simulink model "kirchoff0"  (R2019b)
settings: Solver=ode23s  StartTime=0.0  StopTime=0.01  RelTol=1e-3  EnableMultiTasking=on
libraries: fl_lib x9, nesl_utility x5, powerlib x1

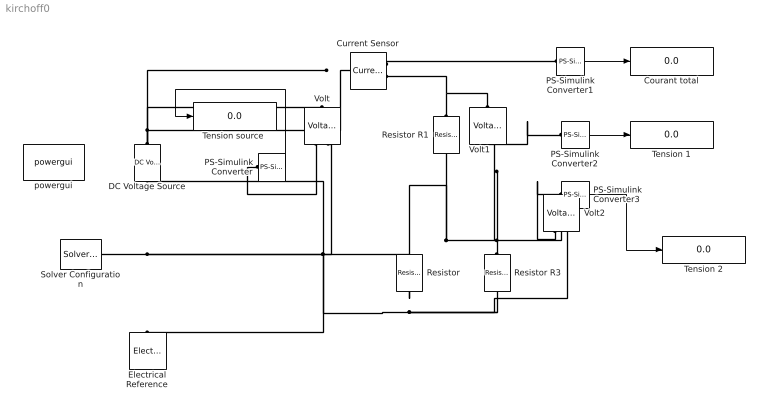
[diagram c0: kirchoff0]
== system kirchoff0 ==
  Courant total : Display
  Current Sensor : fl_lib/Electrical/Electrical Sensors/Current Sensor
  DC Voltage Source : fl_lib/Electrical/Electrical Sources/DC Voltage Source  v0=10 V
  Electrical Reference : fl_lib/Electrical/Electrical Elements/Electrical Reference
  PS-Simulink Converter : nesl_utility/PS-Simulink Converter  PhysicalDomain=network_engine_domain  SubClassName=ps_output  LeftPortType=input  RightPortType=output  PseudoPeriodic=off  Frequencies=[]  Unit=V  AffineConversion=off
  PS-Simulink Converter1 : nesl_utility/PS-Simulink Converter  PhysicalDomain=network_engine_domain  SubClassName=ps_output  LeftPortType=input  RightPortType=output  PseudoPeriodic=off  Frequencies=[]  Unit=A  AffineConversion=off
  PS-Simulink Converter2 : nesl_utility/PS-Simulink Converter  PhysicalDomain=network_engine_domain  SubClassName=ps_output  LeftPortType=input  RightPortType=output  PseudoPeriodic=off  Frequencies=[]  Unit=V  AffineConversion=off
  PS-Simulink Converter3 : nesl_utility/PS-Simulink Converter  PhysicalDomain=network_engine_domain  SubClassName=ps_output  LeftPortType=input  RightPortType=output  PseudoPeriodic=off  Frequencies=[]  Unit=V  AffineConversion=off
  Resistor : fl_lib/Electrical/Electrical Elements/Resistor  R=100 Ohm  i_specify=off  i_priority=None  i=0 A  i_nominal_specify=off  i_nominal_unit=A  i_nominal_value=1  v_specify=off  v_priority=None  v=0 V  v_nominal_specify=off  v_nominal_unit=V  v_nominal_value=1
  Resistor R1 : fl_lib/Electrical/Electrical Elements/Resistor  R=100 Ohm  i_specify=off  i_priority=None  i=0 A  i_nominal_specify=off  i_nominal_unit=A  i_nominal_value=1  v_specify=off  v_priority=None  v=0 V  v_nominal_specify=off  v_nominal_unit=V  v_nominal_value=1
  Resistor R3 : fl_lib/Electrical/Electrical Elements/Resistor  R=100 Ohm  i_specify=off  i_priority=None  i=0 A  i_nominal_specify=off  i_nominal_unit=A  i_nominal_value=1  v_specify=off  v_priority=None  v=0 V  v_nominal_specify=off  v_nominal_unit=V  v_nominal_value=1
  Solver Configuration : nesl_utility/Solver Configuration  PhysicalDomain=network_engine_domain  SubClassName=solver  LeftPortType=input  RightPortType=generic  Tones=[]  Harmonics=[]  SimulateNoise=off  Profile=off  UseLocalSampling=off  EnableSwitchedLinearOptims=on  FrequencyDomain=off  UseCCode=off  RelTol=0.001  AbsTol=1e-06  MinStep=1e-09  ToWorkspace=off  RevertToSquareIcSolve=off  NumHomotopyIterations=100  PhasorMode=off  PhasorModeNumHarmonics=1  DoDC=off  ResidualTolerance=1e-9  UseLocalSolver=off  LocalSolverChoice=NE_BACKWARD_EULER_ADVANCER  LocalSolverSampleTime=.001  DoFixedCost=off  MaxNonlinIter=3  MaxModeIter=2  LinearAlgebra=Sparse  EquationFormulation=NE_TIME_EF  DelaysMemoryBudget=1024  AutomaticFiltering=on  FilteringTimeConstant=0.001  PartitionStorageMethod=AS_NEEDED  PartitionMemoryBudget=1024  PartitionMethod=FAST
  Tension 1 : Display
  Tension 2 : Display
  "Tension source " : Display
  Volt : fl_lib/Electrical/Electrical Sensors/Voltage Sensor
  Volt1 : fl_lib/Electrical/Electrical Sensors/Voltage Sensor
  Volt2 : fl_lib/Electrical/Electrical Sensors/Voltage Sensor
  powergui : powerlib/powergui  Priority=1  SimulationMode=Continuous  SampleTime=50e-6  frequency=60  Iterations=50  frequencyindice=17  Pbase=100e6  ErrMax=1e-4  UnitsV=V  UnitsW=W  buscounter=0  FunctionMessages=off  echomessages=off  EnableUseOfTLC=off  CurrentSourceSwitches=on  DisableSnubberDevices=off  DisableRonSwitches=off  DisableVfSwitches=off  DisplayEquations=off  AutomaticDiscreteSolvers=off  SolverType=Tustin  Interpol=off  ExternalGateDelay=off  methode=off  Ts=100  x0status=blocks  SPID=off  SwTol=0  HookPort=off  NonlinearTolerance=1e-4  nMaxIteration=100  ContinueOnMaxIteration=off  RestoreLinks=warning  ResistiveCurrentMeasurement=off  Frange=[0:2:500]  Ylog=off  Xlog=on  ShowGrid=off  save=off  variable=ZData  structure=0  ZoomFFT=off  StartTime=0.0  cycles=1  DisplayStyle=1  fundamental=60  FreqAxis=off  MaxFrequency=1000  frequencyindicesteady=1  RmsSteady=1  display=off
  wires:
  PS-Simulink Converter1/1 -> Courant total/1
  PS-Simulink Converter/1 -> "Tension source "/1
  PS-Simulink Converter2/1 -> Tension 1/1
  PS-Simulink Converter3/1 -> Tension 2/1
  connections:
  Solver Configuration/RConn1 -- Electrical Reference/LConn1 -- DC Voltage Source/RConn1 -- Volt2/RConn2 -- Resistor R3/RConn1 -- Resistor/RConn1 -- Volt/RConn2
  DC Voltage Source/LConn1 -- Volt/LConn1 -- Current Sensor/LConn1
  Current Sensor/RConn1 -- PS-Simulink Converter1/LConn1
  Resistor R1/LConn1 -- Current Sensor/RConn2 -- Volt1/LConn1
  Volt/RConn1 -- PS-Simulink Converter/LConn1
  Volt1/RConn1 -- PS-Simulink Converter2/LConn1
  Volt2/RConn1 -- PS-Simulink Converter3/LConn1
  Resistor R3/LConn1 -- Resistor/LConn1 -- Resistor R1/RConn1 -- Volt1/RConn2 -- Volt2/LConn1
